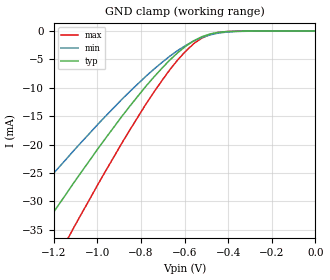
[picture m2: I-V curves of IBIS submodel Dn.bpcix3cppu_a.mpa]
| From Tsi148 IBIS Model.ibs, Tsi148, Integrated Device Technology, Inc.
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[Submodel]  Dn.bpcix3cppu_a.mpa
Submodel_type   Dynamic_clamp
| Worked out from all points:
|   GND clamp passes 1 mA (typ) near -0.52 V on its own axis
[GND Clamp]   | Note: Vtable =  Vout
| Voltage   I(typ)   I(min)   I(max)
-3.6V     -178.7mA   -141.7mA   -221.1mA
-1.437V   -45.52mA   -35.65mA   -58.2mA
-1.4V     -43.37mA   -33.98mA   -55.52mA
-1.253V   -34.89mA   -27.37mA   -44.9mA
-1.143V   -28.68mA   -22.56mA   -37.08mA
-1.107V   -26.64mA   -20.98mA   -34.51mA
-777mV    -9.688mA   -7.935mA   -12.84mA
-667mV    -5.062mA   -4.389mA   -6.752mA
-557mV    -1.681mA   -1.72mA    -2.178mA
-483mV    -506uA     -664uA     -585uA
-410mV    -101uA     -189uA     -92uA
0V        0A         0A         0A
